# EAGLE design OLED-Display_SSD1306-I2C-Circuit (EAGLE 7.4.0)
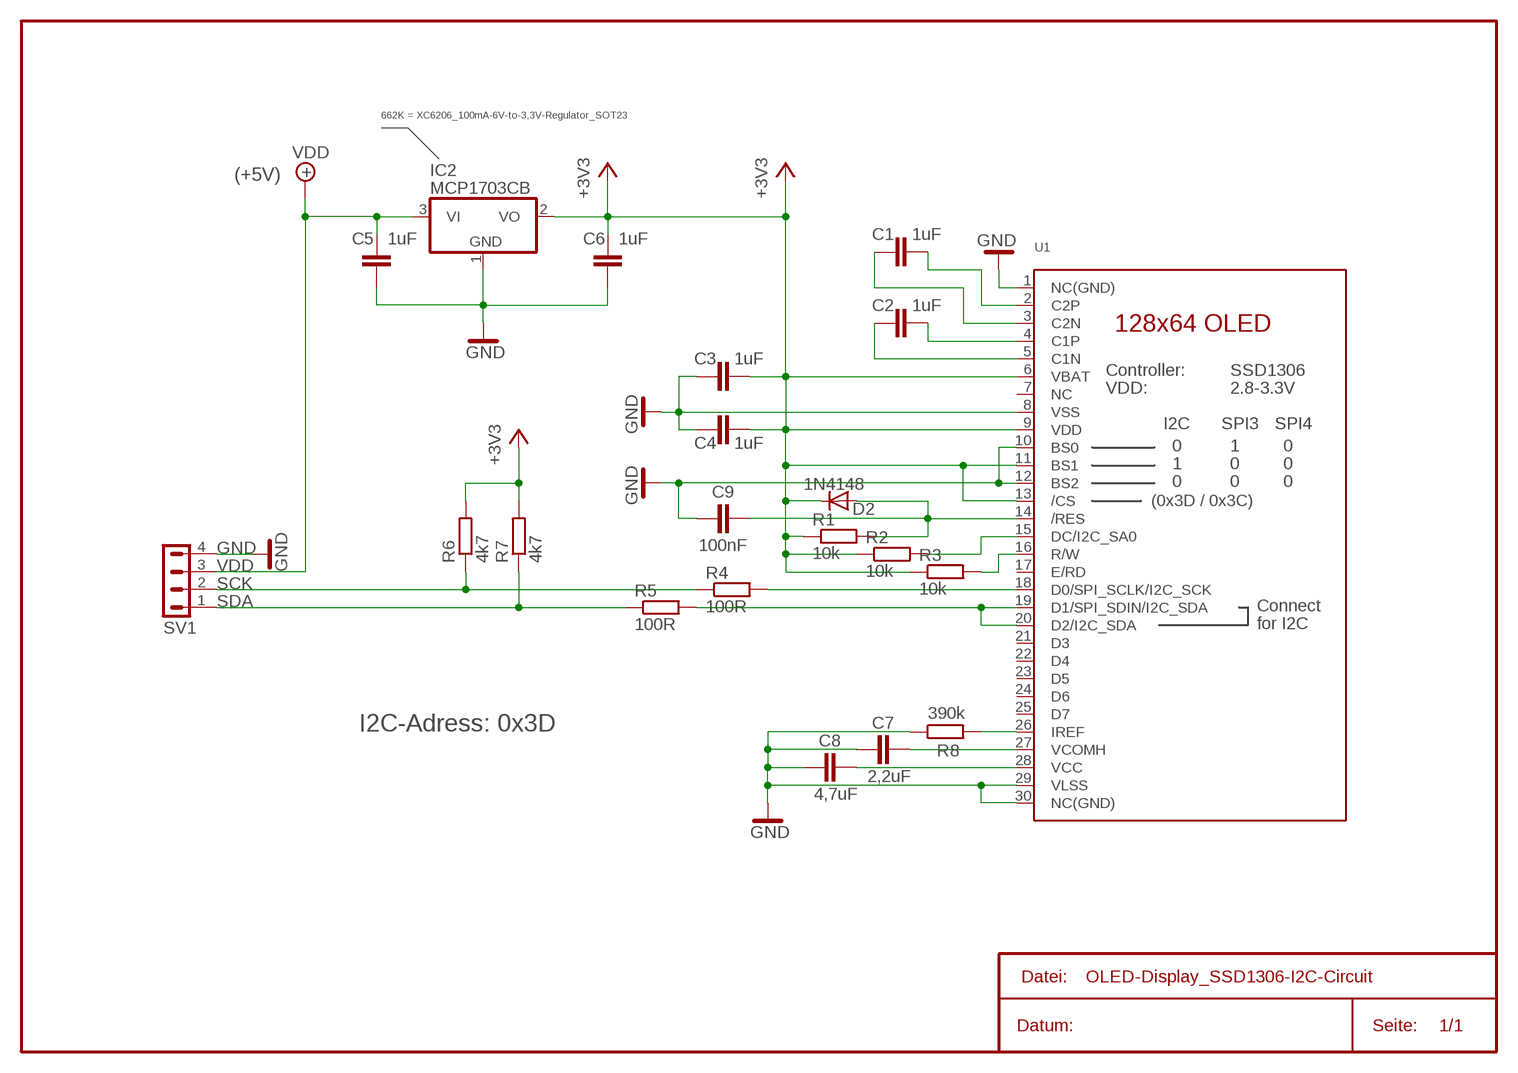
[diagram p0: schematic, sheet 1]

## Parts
C1  1uF  C-EUC0603  [C0603]
C2  1uF  C-EUC0603  [C0603]
C3  1uF  C-EUC0603  [C0603]
C4  1uF  C-EUC0603  [C0603]
C5  1uF  C-EUC0603  [C0603]
C6  1uF  C-EUC0603  [C0603]
C7  2,2uF  C-EUC0603  [C0603]
C8  4,7uF  C-EUC0603  [C0603]
C9  100nF  C-EUC0603  [C0603]
D2  1N4148  DIODE-SOD523  [SOD523]
IC2  MCP1703CB  [SOT23]
R1  10k  R-EU_R0603  [R0603]
R2  10k  R-EU_R0603  [R0603]
R3  10k  R-EU_R0603  [R0603]
R4  100R  R-EU_R0603  [R0603]
R5  100R  R-EU_R0603  [R0603]
R6  4k7  R-EU_R0603  [R0603]
R7  4k7  R-EU_R0603  [R0603]
R8  390k  R-EU_R0603  [R0603]
SV1  MA04-11  [MA04-1R]
U1  DISP_OLED_UG-2864HSWEG010.96"  [UG-2864HSWEG01_0.96IN_WRAPAROUND]

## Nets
+3V3: C3.2 C4.2 C6.2 D2.C IC2.2(VO) R1.1 R2.1 R3.1 R6.2 R7.2 U1.6(VBAT) U1.9(VDD) U1.11(BS1) U1.13(/CS)
GND: C3.1 C4.1 C5.1 C6.1 C7.1 C8.1 C9.1 IC2.1(GND) R8.1 SV1.4 U1.1(NC(GND)) U1.8(VSS) U1.10(BS0) U1.12(BS2) U1.29(VLSS) U1.30(NC(GND))
N$1: C1.2 U1.2(C2P)
N$2: C1.1 U1.3(C2N)
N$3: C2.2 U1.4(C1P)
N$4: C2.1 U1.5(C1N)
N$5: R3.2 U1.16(R/W)
N$6: C9.2 D2.A R1.2 U1.14(/RES)
N$7: R2.2 U1.15(DC/I2C_SA0)
N$8: R4.2 U1.18(D0/SPI_SCLK/I2C_SCK)
N$9: R5.2 U1.19(D1/SPI_SDIN/I2C_SDA) U1.20(D2/I2C_SDA)
N$10: C7.2 U1.27(VCOMH)
N$11: R8.2 U1.26(IREF)
N$13: C8.2 U1.28(VCC)
SCK: R4.1 R6.1 SV1.2
SDA: R5.1 R7.1 SV1.1
VDD: C5.2 IC2.3(VI) SV1.3
Unconnected: U1.7(NC) U1.17(E/RD) U1.21(D3) U1.22(D4) U1.23(D5) U1.24(D6) U1.25(D7)

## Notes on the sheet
- 662K = XC6206_100mA-6V-to-3,3V-Regulator_SOT23
- (+5V) | +
- (0x3D / 0x3C)
- I2C-Adress: 0x3D

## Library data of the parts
C1-C9 = rcl1:C-EU: CAPACITOR, European symbol
D2 = diode1:DIODE-: DIODE
IC2 = linear-2:MCP1703: 250 mA, 16V, Low Quiescent Current LDO Regulator Source: http://ww1.microchip.com/downloads/en/DeviceDoc/22049b.pdf
R1-R8 = rcl1:R-EU_: RESISTOR, European symbol
SV1 = con-lstc:MA04-1: PIN HEADER
U1 = Display-OLED_128x64:DISP_OLED_UG-2864HSWEG01: UG-2864HSWEG01 OLED display Both 1.3" and 0.96" models share the same FPC tab footprint, only the screen dimensions vary.

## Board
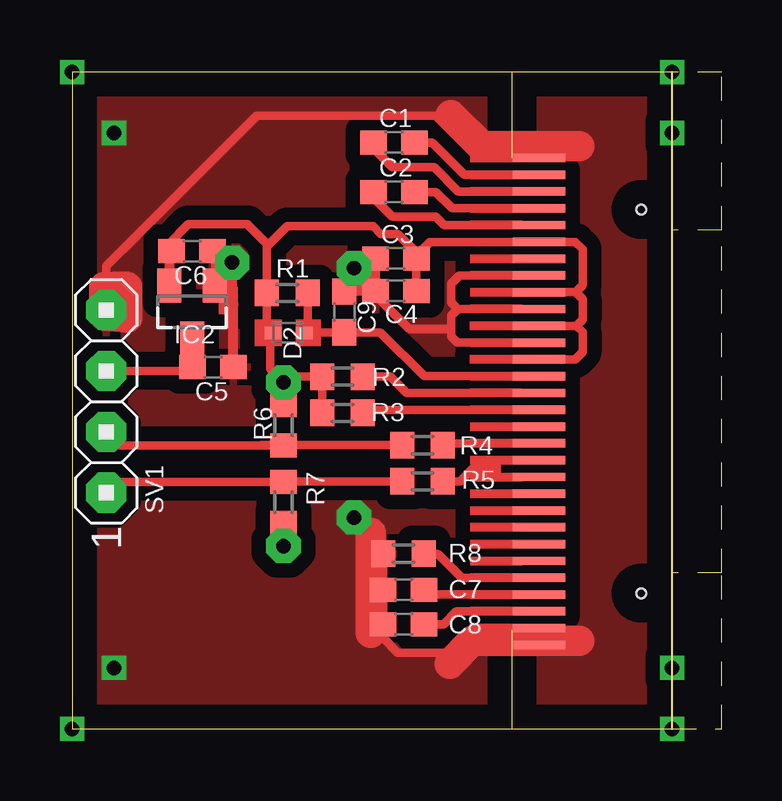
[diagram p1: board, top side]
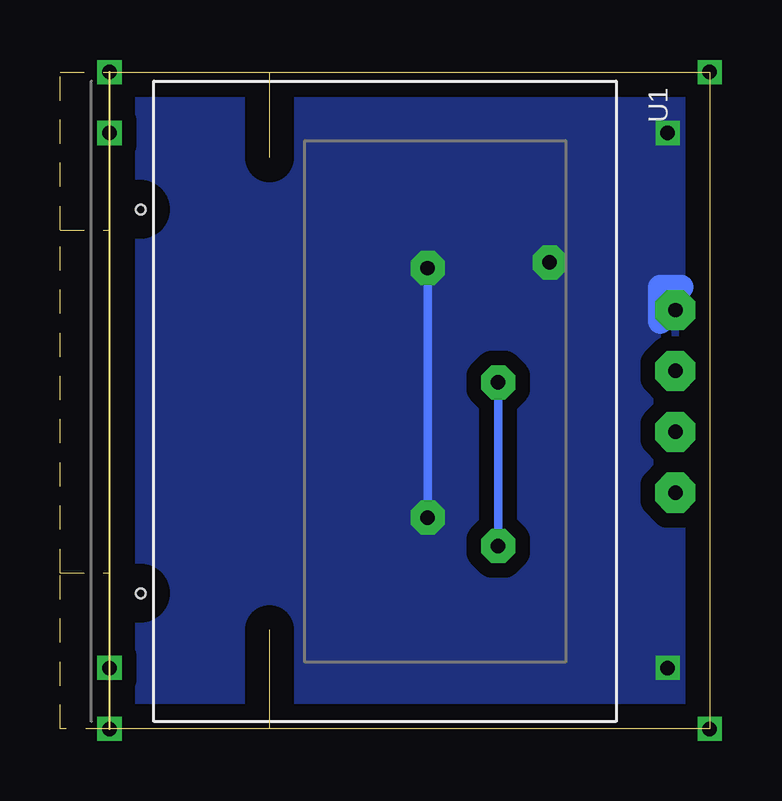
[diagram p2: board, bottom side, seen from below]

Size 27.07 x 27.38 mm. Coordinates in mm from the lower left corner, seen from the top.
Outline: 18.34,0 0,0 0,27.38 18.34,27.38
Outline: 18.34,0 25,0
Outline: 25,0 27.07,0 27.07,6.51
Outline: 25,27.38 27.07,27.38 27.07,20.8
Outline: 25,27.38 18.34,27.38
Outline: 18.34,23.81 18.34,27.38
Outline: 18.34,0 18.34,4.13
Outline: 27.07,6.51 25,6.51
Outline: 25,6.51 25,20.8
Outline: 27.07,20.8 25,20.8
Outline: 25,0 25,6.51
Outline: 25,20.8 25,27.38
Outline: 27.07,6.51 27.07,20.8
Copper layers (1*16): Top 0.035mm / dielectric 1.5mm / Bottom 0.035mm
Design rules "default": minimum track width 10mil, minimum drill 24mil, track to track 8mil, track to pad 8mil, pad to pad 8mil, via to via 8mil, smd to smd 8mil, copper to edge 40mil, drill to drill 8mil, minimum pad ring 10mil, minimum via ring 8mil, stop-mask expansion 4mil, vias tented up to drill 0mil, thermal gap 10mil

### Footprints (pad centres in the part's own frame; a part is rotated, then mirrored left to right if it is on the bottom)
C0603 = smd 1.1 x 1: 1 -0.85,0; 2 0.85,0
SOD523 = smd 0.7 x 0.5: A 0.7,0; C -0.6,0
SOT23 = smd 1 x 1.4: 1 -0.95,-1.1; 2 0.95,-1.1; 3 0,1.1
R0603 = smd 1 x 1.1: 1 -0.85,0; 2 0.85,0
MA04-1R = drill 0.6 pad 1.676 octagon: 1 0,0; 2 2.54,0; 3 5.08,0; 4 7.62,0
UG-2864HSWEG01_0.96IN_WRAPAROUND = smd 0.35 x 2.2 bottom: 1 -10.15,-1.2; 2 -9.45,-1.2; 3 -8.75,-1.2; 4 -8.05,-1.2; 5 -7.35,-1.2; 6 -6.65,-1.2; 7 -5.95,-1.2; 8 -5.25,-1.2; 9 -4.55,-1.2; 10 -3.85,-1.2; 11 -3.15,-1.2; 12 -2.45,-1.2; 13 -1.75,-1.2; 14 -1.05,-1.2; 15 -0.35,-1.2; 16 0.35,-1.2; 17 1.05,-1.2; 18 1.75,-1.2; 19 2.45,-1.2; 20 3.15,-1.2; 21 3.85,-1.2; 22 4.55,-1.2; 23 5.25,-1.2; 24 5.95,-1.2; 25 6.65,-1.2; 26 7.35,-1.2; 27 8.05,-1.2; 28 8.75,-1.2; 29 9.45,-1.2; 30 10.15,-1.2 | hole 0.4: -8,-5.45; 8,-5.45

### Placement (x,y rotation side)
C1  13.41,24.45 0 top
C2  13.41,22.38 0 top
C3  13.49,19.61 0 top
C4  13.49,18.26 0 top
C5  5.87,15.08 180 top
C6  5,19.92 180 top
C7  13.81,5.79 0 top
C8  13.81,4.37 0 top
C9  11.35,17.38 270 top
D2  8.97,16.51 0 top
IC2  5,17.38 180 top
R1  8.97,18.18 0 top
R2  11.27,14.68 0 top
R3  11.27,13.18 0 top
R4  14.61,11.83 0 top
R5  14.61,10.32 0 top
R6  8.81,12.66 90 top
R7  8.81,9.45 270 top
R8  13.81,7.3 0 top
SV1  1.43,9.84 90 top
U1  18.26,13.65 270 bottom

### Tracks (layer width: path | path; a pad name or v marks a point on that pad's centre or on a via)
+3V3  (via drill 0.6 pad 1.42)
  Top 0.356: 14.36,19.59 C3.2 | C4.2 C3.2 | C3.2 14.34,19.87 13.57,20.64 12.86,20.64 12.54,20.95 8.97,20.95 8.18,20.16 | C3.2 14.34,19.74 14.9,20.3 U1.6 20.97,20.3 21.27,20 21.27,18.49 20.98,18.2 | U1.9 20.98,18.2 | 20.98,18.2 21.27,17.91 21.27,17.07 21.01,16.8 | 21.01,16.8 U1.11 | 21.01,16.8 21.27,16.54 21.27,15.72 20.96,15.4 U1.13 | IC2.2 4.04,18.49 | v8.81,14.45 9.05,14.68 R2.1 R3.1 | C6.2 4.04,19.81 4.04,20.23 4.84,21.03 7.3,21.03 8.18,20.16 | v8.81,7.62 R7.2 | 8.18,20.16 8.12,20.11 R1.1 8.12,16.76 D2.C 8.26,16.4 8.26,15 v8.81,14.45 | v8.81,14.45 R6.2
  Top 0.406: 4.04,19.81 4.05,19.81 IC2.2
  Bottom 0.356: v8.81,7.62 v8.81,14.45
GND  (via drill 0.6, 0.6 pad 1.42)
  Top 0: 16.92,23.8 16.84,24.14
  Top 0.356: U1.8 16.12,18.9 15.8,18.57 15.8,17.78 16.03,17.54 16.03,17.46 | U1.10 16.15,17.5 16.03,17.46 | C4.1 C3.1 12.14,19.61 v11.75,19.21 | C4.1 12.64,18.07 14.05,16.67 15.72,16.67 15.8,16.59 | 16.03,17.46 15.8,17.23 15.8,16.59 | 15.8,16.59 15.8,16.35 16.04,16.1 U1.12 | 2.06,18.1 SV1.4 1.43,19.29 7.7,25.56 15.16,25.56 16.92,23.8 U1.1 | C9.1 12.62,18.23 C4.1 | 5.96,19.45 5.96,18.49 IC2.1 6.72,17.71 | 5.96,19.45 5.96,19.81 C6.1 | 12.96,4.39 C7.1 R8.1 | U1.29 U1.30 16.52,3.5 16.19,3.17 13.57,3.17 12.96,3.79 C8.1 12.54,4.76 12.54,8.02 v11.75,8.81 | 5.96,19.45 v6.67,19.45 6.44,19.45 6.36,19.37
  Top 0.406: 12.96,3.79 12.75,4 12.45,4 | 5.98,20.05 C6.1 | C8.1 12.96,4.39 | C5.1 6.72,17.71
  Top 1.016: 6.36,18.41 6.36,19.37
  Top 1.27: 21.12,3.66 16.68,3.66 15.73,2.71 | 12.45,8.18 12.45,4 | 2.3,18.41 1.35,18.41 1.35,17.22 2.3,17.14 2.3,18.37 | 21.12,24.3 17.08,24.3 15.79,25.59
  Bottom 0.356: v11.75,19.21 v11.75,8.81
  Bottom 0.406: 2.06,16.99 1.59,17.46 SV1.4
  Bottom 1.016: 2.06,16.99 2.06,18.41 1.19,18.41
  other vias: 1.75,2.54 1.75,24.84
  pour Top (isolate 0.61): -0.32,27.62 27.3,27.62 27.3,-0.32 -0.32,-0.32
  pour Bottom (isolate 0.61): -0.32,27.62 27.3,27.62 27.3,-0.32 -0.32,-0.32
N$1
  Top 0.356: U1.2 16.35,23.1 15,24.45 C1.2
N$2
  Top 0.356: U1.3 16.09,22.4 15.08,23.42 13.34,23.42 12.56,24.19 C1.1 12.72,24.11
N$3
  Top 0.356: U1.4 15.84,21.7 15.16,22.38 C2.2
N$4
  Top 0.356: U1.5 15.51,21 15.16,21.35 13.34,21.35 12.56,22.12 C2.1
N$5
  Top 0.356: U1.16 12.25,13.3 R3.2
N$6
  Top 0.356: U1.14 14.67,14.7 12.84,16.53 C9.2 9.69,16.53 D2.A 9.82,16.66 R1.2
N$7
  Top 0.356: U1.15 13.94,14 13.26,14.68 R2.2
N$8
  Top 0.356: U1.18 15.54,11.9 R4.2
N$9
  Top 0.356: R5.2 16.17,10.32 16.7,10.85 17.7,10.85 | 17.7,10.85 17.7,11.19 U1.19 | 17.7,10.85 17.7,10.51 U1.20
N$10
  Top 0.356: C7.2 14.85,5.6 U1.27
N$11
  Top 0.356: U1.26 16.24,6.3 15.24,7.3 R8.2
N$12  (via drill 0.6)
  other vias: 25,0
N$13
  Top 0.356: U1.28 16.02,4.9 15.48,4.37 C8.2
N$14  (via drill 0.6)
  other vias: 0,0
N$15  (via drill 0.6)
  other vias: 0,27.38
N$16  (via drill 0.6)
  other vias: 25,27.38
N$17  (via drill 0.6)
  other vias: 25,24.84
N$18  (via drill 0.6)
  other vias: 25,2.54
SCK
  Top 0.356: R4.1 7.88,11.83 R6.1 2,11.81 SV1.2
SDA
  Top 0.356: R5.1 9.07,10.32 R7.1 1.88,10.3 SV1.1
VDD
  Top 0.356: SV1.3 4.87,14.92 C5.2 5.02,16.26 IC2.3
(copper drawn outside any net)
  shapes: Top area x32

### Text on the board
tValues: GND | VDD | SCK | SDA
